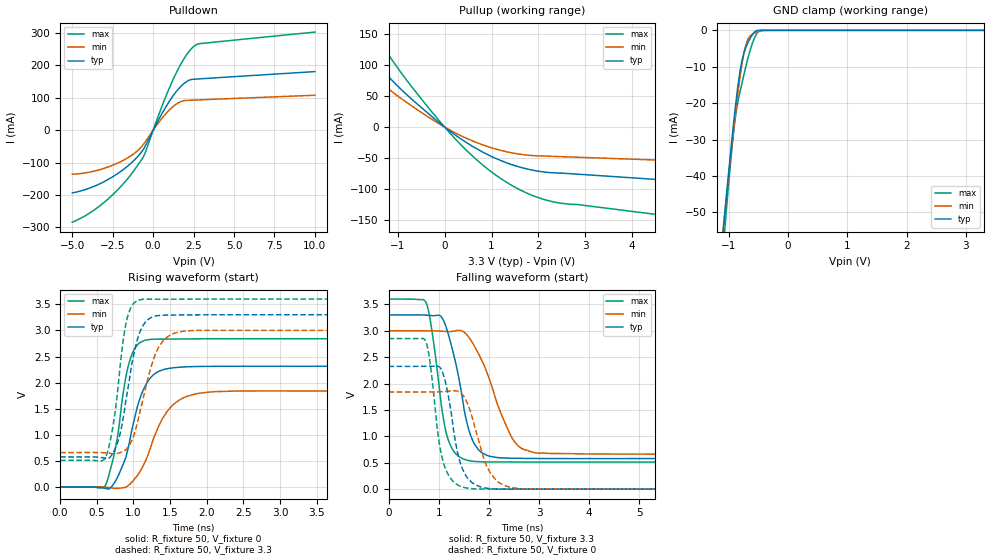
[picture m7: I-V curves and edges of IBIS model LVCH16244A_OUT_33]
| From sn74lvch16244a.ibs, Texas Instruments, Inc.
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[Model]   LVCH16244A_OUT_33
Model_type  3-state
Enable   Active-Low
Vref =   0
Rref =   500
Cref =   50p
Vmeas =   1.5
| variable   typ   min   max
C_comp   4.66pF   4.13pF   6.00pF
| C_pullup   6.54pF   3.89pF   9.70pF
| C_pulldown   6.87pF   5.28pF   8.79pF
| C_tri-state   4.66pF   4.13pF   6.00pF
[Temperature Range]   40   100   -40
| Ambient temperature   25   85   -40
[Voltage range]   3.3   3   3.6
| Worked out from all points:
|   slope of the pulldown table from 0 to 0.495 V, typ, clamps not added: 10.5 ohm
|   slope of the pullup table from 0 to 0.495 V, typ, clamps not added: 18.7 ohm
|   GND clamp passes 1 mA (typ) near -0.59 V on its own axis
|   rising waveform, R_fixture 50, V_fixture 0: 20-80 % time 265ps typ, 355ps min, 194ps max; typ from 0 V to 2.31 V
|   falling waveform, R_fixture 50, V_fixture 3.3: 20-80 % time 358ps typ, 570ps min, 266ps max; typ from 3.3 V to 0.578 V
|   rising waveform, R_fixture 50, V_fixture 3.3: 20-80 % time 207ps typ, 261ps min, 163ps max; typ from 0.578 V to 3.3 V
|   falling waveform, R_fixture 50, V_fixture 0: 20-80 % time 269ps typ, 362ps min, 231ps max; typ from 2.32 V to 0 V
[GND Clamp]
| LVCH16244A_OUT_33
|   Voltage   I(typ)   I(min)   I(max)
-5V       -855.7mA   -797.6mA   -953.2mA
-1.095V   -55.25mA   -54.79mA   -60.22mA
-1.065V   -49.94mA   -49.9mA    -54.27mA
-955mV    -31.29mA   -32.66mA   -33.81mA
-910mV    -24.24mA   -26.03mA   -26.76mA
-860mV    -17.12mA   -19.11mA   -20.92mA
-795mV    -9.817mA   -11.17mA   -15.81mA
-735mV    -5.784mA   -5.591mA   -11.55mA
-680mV    -3.534mA   -2.583mA   -7.881mA
-580mV    -736.5uA   -852.5uA   -2.652mA
-485mV    -14.03uA   -258.5uA   -126.7uA
3.3V      10.95pA    55.96nA    -30.28pA
[Pulldown]
| LVCH16244A_OUT_33
|   Voltage   I(typ)   I(min)   I(max)
-5V       -193.4mA   -135.8mA   -283.8mA
-3.87V    -177.4mA   -128.6mA   -253.7mA
-2.72V    -150.1mA   -112.1mA   -209.2mA
-1.54V    -109.1mA   -84.13mA   -147.4mA
-730mV    -67.77mA   -51.47mA   -92.05mA
-485mV    -48.43mA   -35.35mA   -68.52mA
485mV     46.17mA    33.18mA    66.28mA
1.245V    107.2mA    73.64mA    157.8mA
1.945V    145.9mA    91.78mA    224mA
2.535V    157.6mA    93.17mA    259.6mA
2.87V     158.7mA    93.86mA    267.5mA
10V       181.2mA    108.1mA    303.1mA
[Pullup]
| LVCH16244A_OUT_33
|   Voltage   I(typ)   I(min)   I(max)
-5V       388.2mA    115.6mA    569.5mA
-4.8V     377.1mA    131.8mA    547.8mA
-4.67V    368.8mA    170.1mA    533.4mA
-2.73V    213.4mA    164.5mA    302.6mA
-2.425V   186.8mA    144.1mA    265.2mA
-1.63V    117.9mA    90.44mA    167.3mA
-735mV    47.21mA    35.83mA    68.13mA
480mV     -25.67mA   -18.52mA   -38.57mA
1.275V    -56.24mA   -38.95mA   -86.83mA
2.13V     -72.49mA   -46.66mA   -117mA
6.525V    -94.6mA    -58.57mA   -160mA
10V       -112.3mA   -68.03mA   -193.4mA
[Ramp]
| LVCH16244A_OUT_33
| variable   typ   min   max
dV/dt_r   1.41/2.74E-10   1.12/3.67E-10   1.72/2.00E-10
dV/dt_f   1.63/3.65E-10   1.41/5.87E-10   1.85/2.70E-10
R_load = 50
[Rising Waveform]
| LVCH16244A_OUT_33
R_fixture =   50
C_fixture =   0
L_fixture =   0
V_fixture =   0
V_fixture_min = 0
V_fixture_max = 0
|   Time   V(typ)   V(min)   V(max)
0s        -16.98uV   -36.16uV   -6.412uV
610ps     -21.93mV   1.852mV    17.62mV
750ps     105.4mV    -24.29mV   716.8mV
885ps     530.2mV    -4.85mV    2.018V
960ps     966.7mV    69.88mV    2.466V
1.095ns   1.723V     312.1mV    2.772V
1.255ns   2.128V     849.8mV    2.83V
1.635ns   2.296V     1.674V     2.836V
2.395ns   2.315V     1.84V      2.841V
50ns      2.314V     1.838V     2.84V
[Falling Waveform]
| LVCH16244A_OUT_33
R_fixture =   50
C_fixture =   0
L_fixture =   0
V_fixture =   3.3
V_fixture_min = 3
V_fixture_max = 3.6
|   Time   V(typ)   V(min)   V(max)
0s        3.3V       3V         3.6V
745ps     3.296V     3V         3.543V
870ps     3.285V     2.998V     2.971V
1.065ns   3.247V     2.991V     1.507V
1.295ns   2.565V     2.993V     724.9mV
1.565ns   1.249V     2.92V      547.2mV
1.745ns   809.4mV    2.652V     521.4mV
2.465ns   584mV      962.7mV    513mV
2.985ns   579.3mV    680.8mV    512.6mV
50ns      578mV      661.9mV    512.8mV
[Rising Waveform]
| LVCH16244A_OUT_33
R_fixture =   50
C_fixture =   0
L_fixture =   0
V_fixture =   3.3
V_fixture_min = 3
V_fixture_max = 3.6
|   Time   V(typ)   V(min)   V(max)
0s        578mV      661.8mV    512.8mV
610ps     558.1mV    657.1mV    538.1mV
695ps     598.3mV    644.8mV    972.3mV
775ps     825.9mV    644.6mV    1.726V
910ps     1.769V     736mV      3.208V
1.03ns    2.698V     1.106V     3.55V
1.135ns   3.101V     1.714V     3.597V
1.395ns   3.29V      2.784V     3.597V
1.875ns   3.298V     3.001V     3.599V
50ns      3.3V       3V         3.6V
[Falling Waveform]
| LVCH16244A_OUT_33
R_fixture =   50
C_fixture =   0
L_fixture =   0
V_fixture =   0
V_fixture_min = 0
V_fixture_max = 0
|   Time   V(typ)   V(min)   V(max)
0s        2.324V     1.84V      2.852V
745ps     2.327V     1.84V      2.795V
830ps     2.327V     1.84V      2.385V
1.03ns    2.3V       1.845V     767.4mV
1.165ns   1.896V     1.852V     321.7mV
1.415ns   548.5mV    1.843V     61.05mV
1.705ns   95.68mV    1.233V     4.767mV
2.12ns    1.51mV     196.8mV    706.7uV
2.815ns   45.8uV     1.334mV    34.25uV
50ns      6.233uV    25.44uV    3.464uV
